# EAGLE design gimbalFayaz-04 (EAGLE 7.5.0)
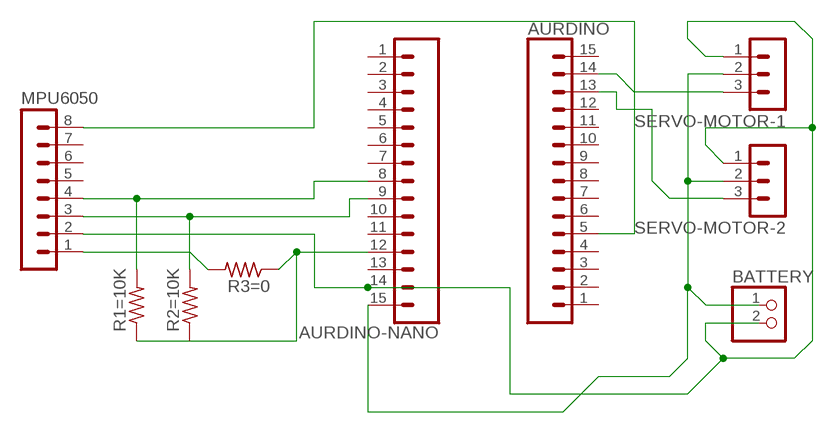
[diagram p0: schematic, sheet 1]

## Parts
AURDINO  CONN_15  [1X15]
AURDINO-NANO  CONN_15  [1X15]
BATTERY  PINHD-1X2  [1X02]
MPU6050  MA08-1  [MA08-1]
R1=10K  RES-US1206FAB  [R1206FAB]
R2=10K  RES-US1206FAB  [R1206FAB]
R3=0  RES-US1206FAB  [R1206FAB]
SERVO-MOTOR-1  MA03-1  [MA03-1]
SERVO-MOTOR-2  MA03-1  [MA03-1]

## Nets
5V: AURDINO-NANO.15 BATTERY.1 SERVO-MOTOR-1.2 SERVO-MOTOR-2.2
D10: AURDINO.13 SERVO-MOTOR-2.3
D11: AURDINO.14 SERVO-MOTOR-1.3
GND: AURDINO-NANO.14 BATTERY.2 MPU6050.2 SERVO-MOTOR-1.1 SERVO-MOTOR-2.1
N$1: MPU6050.1 R3=0.2
N$4: AURDINO-NANO.9 MPU6050.3 R2=10K.2
N$6: AURDINO-NANO.8 MPU6050.4 R1=10K.2
N$7: AURDINO.5 MPU6050.8
N$9: AURDINO-NANO.12 R1=10K.1 R2=10K.1 R3=0.1
Unconnected: AURDINO-NANO.1 AURDINO-NANO.2 AURDINO-NANO.3 AURDINO-NANO.4 AURDINO-NANO.5 AURDINO-NANO.6 AURDINO-NANO.7 AURDINO-NANO.10 AURDINO-NANO.11 AURDINO-NANO.13 AURDINO.1 AURDINO.2 AURDINO.3 AURDINO.4 AURDINO.6 AURDINO.7 AURDINO.8 AURDINO.9 AURDINO.10 AURDINO.11 AURDINO.12 AURDINO.15 MPU6050.5 MPU6050.6 MPU6050.7

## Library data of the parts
AURDINO AURDINO-NANO = SparkFun-Connectors:CONN_15: Multi connection point. Often used as Generic Header-pin footprint for 0.1 inch spaced/style header connections On any of the 0.1 inch spaced packages, you can populate with these: Break Away Headers - Straight (PRT-00116) Break Away Male Headers - Right Angle (PRT-00553) Female Headers (PRT-00115)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
BATTERY = pinhead:PINHD-1X2: PIN HEADER
MPU6050 = con-lstb:MA08-1: PIN HEADER; OC_FARNELL: unknown; OC_NEWARK: unknown
R1=10K R2=10K R3=0 = fab:RES-US: Resistor (US Symbol)
SERVO-MOTOR-1 SERVO-MOTOR-2 = con-lstb:MA03-1: PIN HEADER; OC_FARNELL: unknown; OC_NEWARK: unknown

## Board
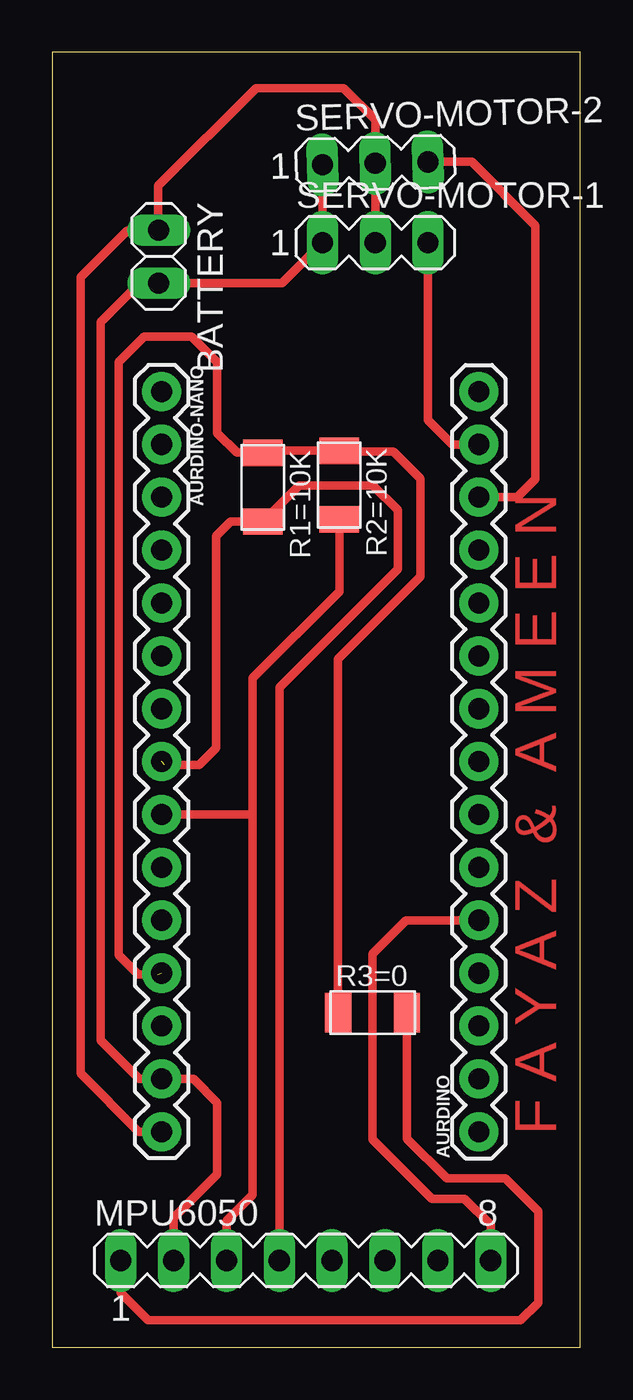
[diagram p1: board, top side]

Size 25.4 x 62.23 mm. Coordinates in mm from the lower left corner, seen from the top.
Outline: 0,0 25.4,0 25.4,62.23 0,62.23 0,0
Copper layers (1*16): Top 0.035mm / dielectric 1.5mm / Bottom 0.035mm
Design rules "default": minimum track width 10mil, minimum drill 24mil, track to track 8mil, track to pad 8mil, pad to pad 8mil, via to via 8mil, smd to smd 8mil, copper to edge 40mil, drill to drill 8mil, minimum pad ring 10mil, minimum via ring 8mil, stop-mask expansion 4mil, vias tented up to drill 0mil, thermal gap 10mil

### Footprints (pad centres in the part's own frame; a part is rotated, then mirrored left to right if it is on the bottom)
1X15 = drill 1.016 pad 1.88: 1 0,0; 2 2.54,0; 3 5.08,0; 4 7.62,0; 5 10.16,0; 6 12.7,0; 7 15.24,0; 8 17.78,0; 9 20.32,0; 10 22.86,0; 11 25.4,0; 12 27.94,0; 13 30.48,0; 14 33.02,0; 15 35.56,0
1X02 = drill 1.016 long: 1 -1.27,0; 2 1.27,0
MA08-1 = drill 1.016 long: 1 -8.89,0; 2 -6.35,0; 3 -3.81,0; 4 -1.27,0; 5 1.27,0; 6 3.81,0; 7 6.35,0; 8 8.89,0
R1206FAB = smd 1.27 x 1.905: 1 -1.651,0; 2 1.651,0
MA03-1 = drill 1.016 long: 1 -2.54,0; 2 0,0; 3 2.54,0

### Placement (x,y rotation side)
AURDINO  20.51,10.36 90 top
AURDINO-NANO  5.27,45.92 270 top
BATTERY  5.13,52.4 270 top
MPU6050  12.19,4.18 0 top
R1=10K  10.13,41.33 270 top
R2=10K  13.8,41.43 270 top
R3=0  15.41,16.09 0 top
SERVO-MOTOR-1  15.53,53.07 0 top
SERVO-MOTOR-2  15.53,56.88 1.6 top

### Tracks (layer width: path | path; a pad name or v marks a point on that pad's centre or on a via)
5V
  Top 0.406: SERVO-MOTOR-1.2 SERVO-MOTOR-2.2 15.53,58.98 14.01,60.5 9.8,60.5 5.11,55.8 5.11,53.7 BATTERY.1 5.11,53.65 3.61,53.65 1.37,51.41 1.37,13.16 4.17,10.36 AURDINO-NANO.15
D10
  Top 0.406: SERVO-MOTOR-2.3 20.17,56.95 23.23,53.89 23.23,41.71 22.36,40.84 AURDINO.13
D11
  Top 0.406: AURDINO.14 19.24,43.38 18.07,44.55 SERVO-MOTOR-1.3
GND
  Top 0.406: MPU6050.2 5.84,6.22 7.94,8.32 7.94,11.76 6.79,12.9 AURDINO-NANO.14 4.19,12.9 2.35,14.74 2.35,49.26 4.24,51.16 5.11,51.16 BATTERY.2 11.05,51.13 SERVO-MOTOR-1.1 SERVO-MOTOR-2.1
N$1
  Top 0.406: MPU6050.1 3.3,2.62 4.62,1.29 22.52,1.29 23.37,2.15 23.37,6.54 21.79,8.12 18.97,8.12 17.06,10.03 R3=0.2
N$4
  Top 0.406: R2=10K.2 13.8,36.32 9.64,32.16 9.64,25.73 | AURDINO-NANO.9 9.51,25.6 9.64,25.73 | MPU6050.3 8.38,6.08 9.64,7.34 9.64,25.73
N$6  (1 unrouted)
  Top 0.406: 5.41,27.98 7.06,27.98 7.87,28.79 7.87,38.98 8.57,39.67 R1=10K.2 11.87,41.41 15.43,41.41 16.62,40.22 16.62,37.4 10.92,31.7 MPU6050.4
N$7
  Top 0.406: MPU6050.8 21.08,5.88 19.81,7.15 18.25,7.15 15.4,9.99 15.4,18.91 17.02,20.52 AURDINO.5
N$9  (1 unrouted)
  Top 0.406: R3=0.1 13.75,33.07 17.72,37.03 17.72,41.73 16.41,43.04 13.84,43.04 R2=10K.1 10.24,43.08 R1=10K.1 8.89,42.98 7.94,43.93 7.94,47.33 6.72,48.55 4.42,48.55 3.21,47.35 3.21,18.85 4.14,17.92 5.08,17.92

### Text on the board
Top: F A Y A Z & A M E E N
